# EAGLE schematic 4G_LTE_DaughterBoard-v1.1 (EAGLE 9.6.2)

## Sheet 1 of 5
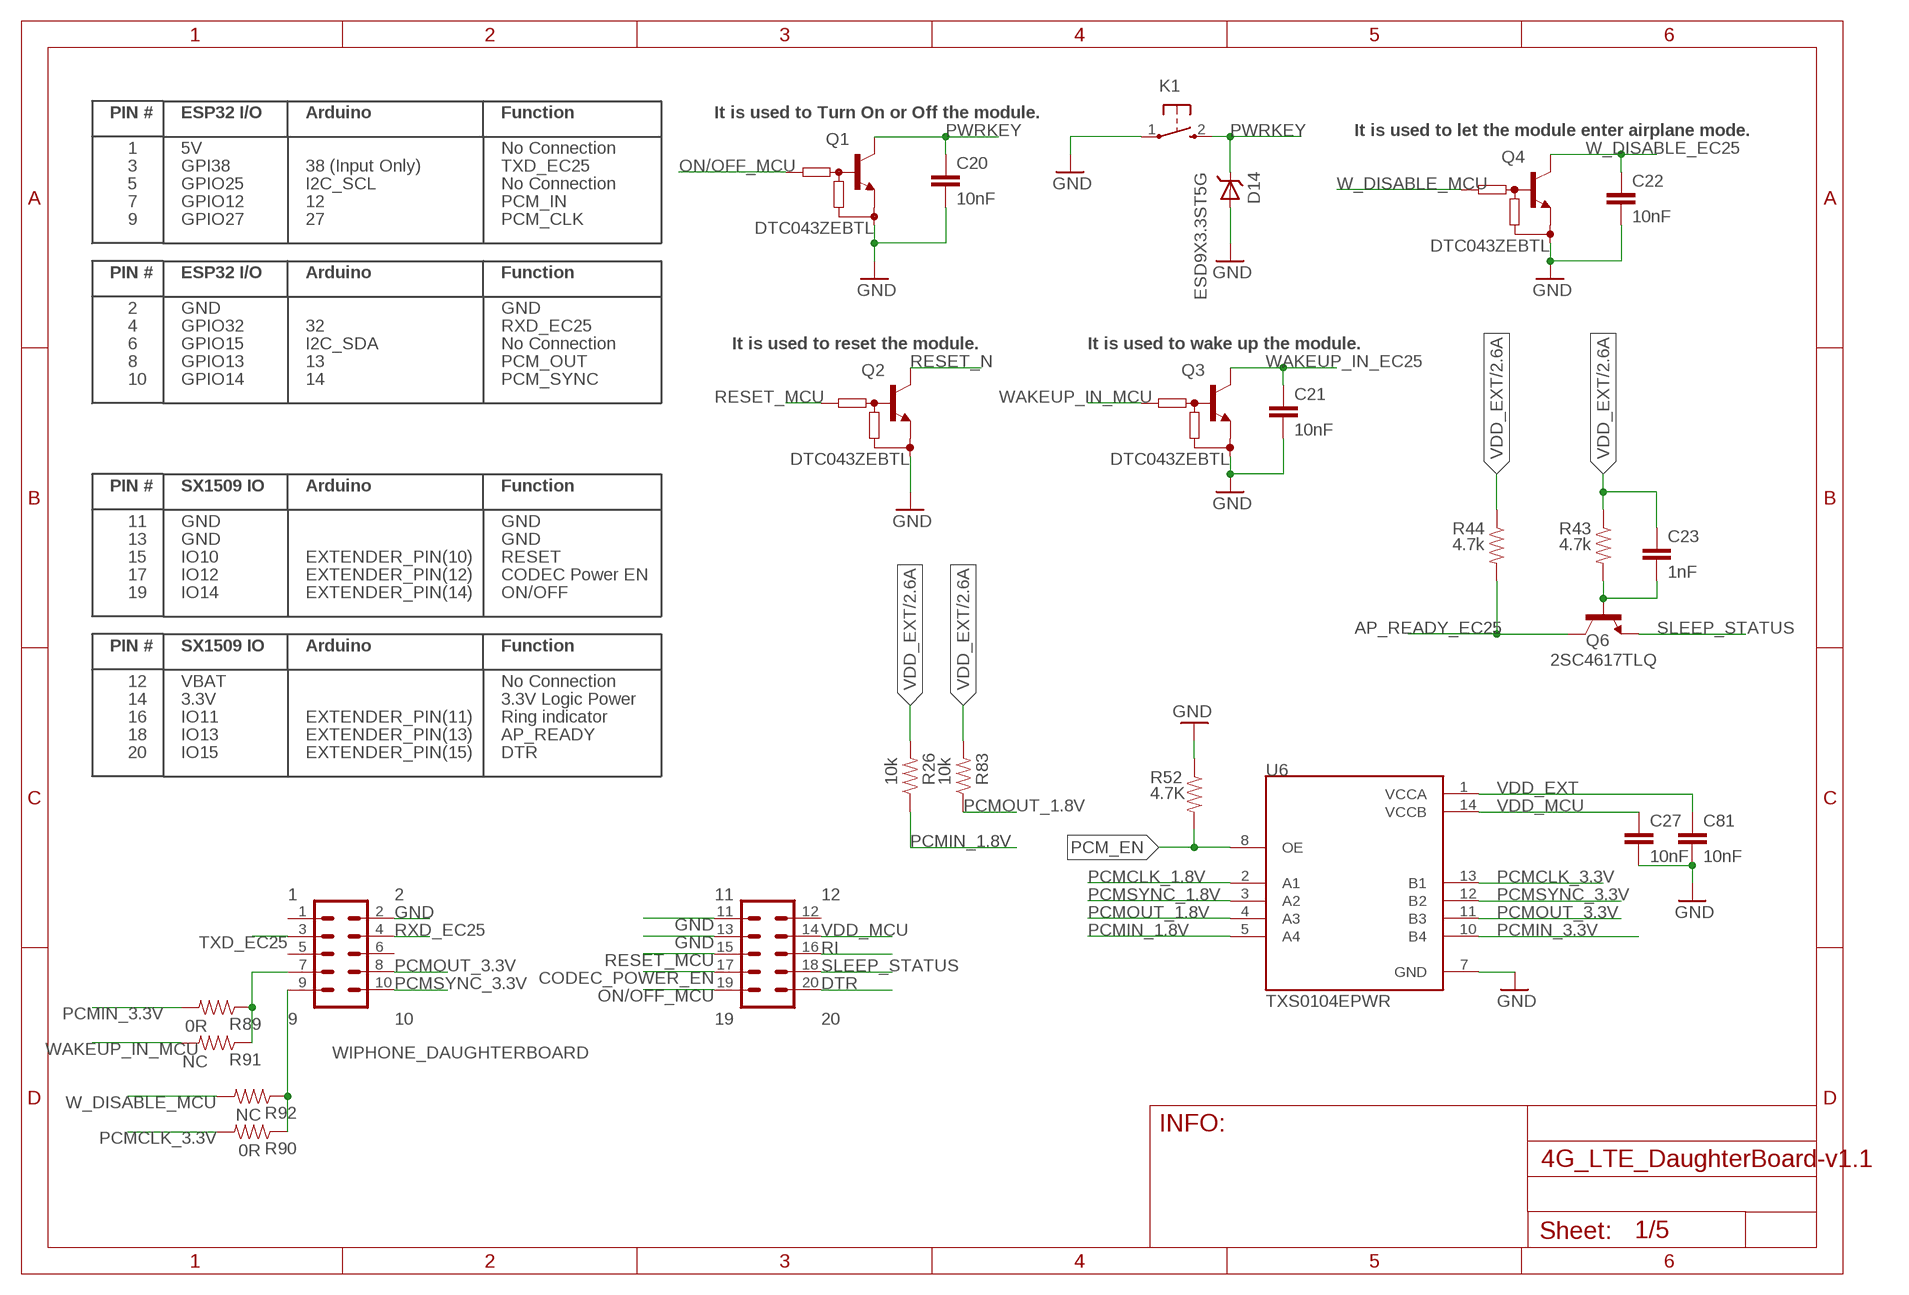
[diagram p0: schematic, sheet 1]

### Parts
C20  10nF  CAP0402  [0402-CAP]
C21  10nF  CAP0402  [0402-CAP]
C22  10nF  CAP0402  [0402-CAP]
C23  1nF  CAP0402  [0402-CAP]
C27  10nF  CAP0402  [0402-CAP]
C81  10nF  CAP0402  [0402-CAP]
D14  ESD9X3.3ST5G  [SODFL1060X40N]
K1  BUTTON_3X6X5-90_DEGREE  [3X6X5-90_DEGREE]
Q1  DTC043ZEBTL  DIGITAL_TRANSISTOR-SC89  [SC89]
Q2  DTC043ZEBTL  DIGITAL_TRANSISTOR-SC89  [SC89]
Q3  DTC043ZEBTL  DIGITAL_TRANSISTOR-SC89  [SC89]
Q4  DTC043ZEBTL  DIGITAL_TRANSISTOR-SC89  [SC89]
Q6  2SC4617TLQ  TRANS_NPN-L  [SOT23-3-L]
R26  10k  RES0402  [0402-RES]
R43  4.7k  RES0402  [0402-RES]
R44  4.7k  RES0402  [0402-RES]
R52  4.7K  RES0402  [0402-RES]
R83  10k  RES0402  [0402-RES]
R89  0R  RES0402  [0402-RES]
R90  0R  RES0402  [0402-RES]
R91  NC  RES0402  [0402-RES]
R92  NC  RES0402  [0402-RES]
U6  TXS0104EPWR  [SOP65P640X120-14N]
WIPHONE_DAUGHTERBOARD-FOOTPRINT1  WIPHONE_DAUGHTERBOARD  [WIPHONE_DAUGHTERBOARD]

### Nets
AP_READY_EC25: Q6.3(C) R44.2 ; also sheet 2
CODEC_POWER_EN: WIPHONE_DAUGHTERBOARD-FOOTPRINT1.17 ; also sheet 5
DTR: WIPHONE_DAUGHTERBOARD-FOOTPRINT1.20 ; also sheet 2
GND: C20.2 C21.2 C22.2 C27.2 C81.2 D14.2 K1.1 Q1.2(E) Q2.2(E) Q3.2(E) Q4.2(E) R52.1 U6.7(GND) WIPHONE_DAUGHTERBOARD-FOOTPRINT1.2 WIPHONE_DAUGHTERBOARD-FOOTPRINT1.11 WIPHONE_DAUGHTERBOARD-FOOTPRINT1.13 ; also sheet 2,3,4,5
N$29: C23.2 Q6.1(B) R43.2
N$73: R89.1 R91.1 WIPHONE_DAUGHTERBOARD-FOOTPRINT1.7
N$74: R90.1 R92.1 WIPHONE_DAUGHTERBOARD-FOOTPRINT1.9
ON/OFF_MCU: Q1.1(B) WIPHONE_DAUGHTERBOARD-FOOTPRINT1.19
PCM_EN: R52.2 U6.8(OE)
PCMCLK_1.8V: U6.2(A1) ; also sheet 2
PCMCLK_3.3V: R90.2 U6.13(B1)
PCMIN_1.8V: R26.1 U6.5(A4) ; also sheet 2
PCMIN_3.3V: R89.2 U6.10(B4)
PCMOUT_1.8V: R83.1 U6.4(A3) ; also sheet 2
PCMOUT_3.3V: U6.11(B3) WIPHONE_DAUGHTERBOARD-FOOTPRINT1.8
PCMSYNC_1.8V: U6.3(A2) ; also sheet 2
PCMSYNC_3.3V: U6.12(B2) WIPHONE_DAUGHTERBOARD-FOOTPRINT1.10
PWRKEY: C20.1 D14.1 K1.2 Q1.3(C) ; also sheet 2
RESET_MCU: Q2.1(B) WIPHONE_DAUGHTERBOARD-FOOTPRINT1.15
RESET_N: Q2.3(C) ; also sheet 2
RI: WIPHONE_DAUGHTERBOARD-FOOTPRINT1.16 ; also sheet 2
RXD_EC25: WIPHONE_DAUGHTERBOARD-FOOTPRINT1.4 ; also sheet 2
SLEEP_STATUS: Q6.2(E) WIPHONE_DAUGHTERBOARD-FOOTPRINT1.18
TXD_EC25: WIPHONE_DAUGHTERBOARD-FOOTPRINT1.3 ; also sheet 2
VDD_EXT: C23.1 C81.1 R26.2 R43.1 R44.1 R83.2 U6.1(VCCA) ; also sheet 2,3,5
VDD_MCU: C27.1 U6.14(VCCB) WIPHONE_DAUGHTERBOARD-FOOTPRINT1.14
W_DISABLE_EC25: C22.1 Q4.3(C) ; also sheet 2
W_DISABLE_MCU: Q4.1(B) R92.2
WAKEUP_IN_EC25: C21.1 Q3.3(C) ; also sheet 2
WAKEUP_IN_MCU: Q3.1(B) R91.2
Unconnected: WIPHONE_DAUGHTERBOARD-FOOTPRINT1.5 WIPHONE_DAUGHTERBOARD-FOOTPRINT1.6

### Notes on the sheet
- It is used to Turn On or Off the module.
- It is used to let the module enter airplane mode.
- No Connection
- TXD_EC25
- No Connection
- PCM_IN
- PCM_CLK
- GND
- RXD_EC25
- No Connection | It is used to reset the module. | It is used to wake up the module.
- PCM_OUT
- PCM_SYNC
- GND
- GND
- RESET
- CODEC Power EN
- ON/OFF
- No Connection
- 3.3V Logic Power
- Ring indicator
- AP_READY
- DTR

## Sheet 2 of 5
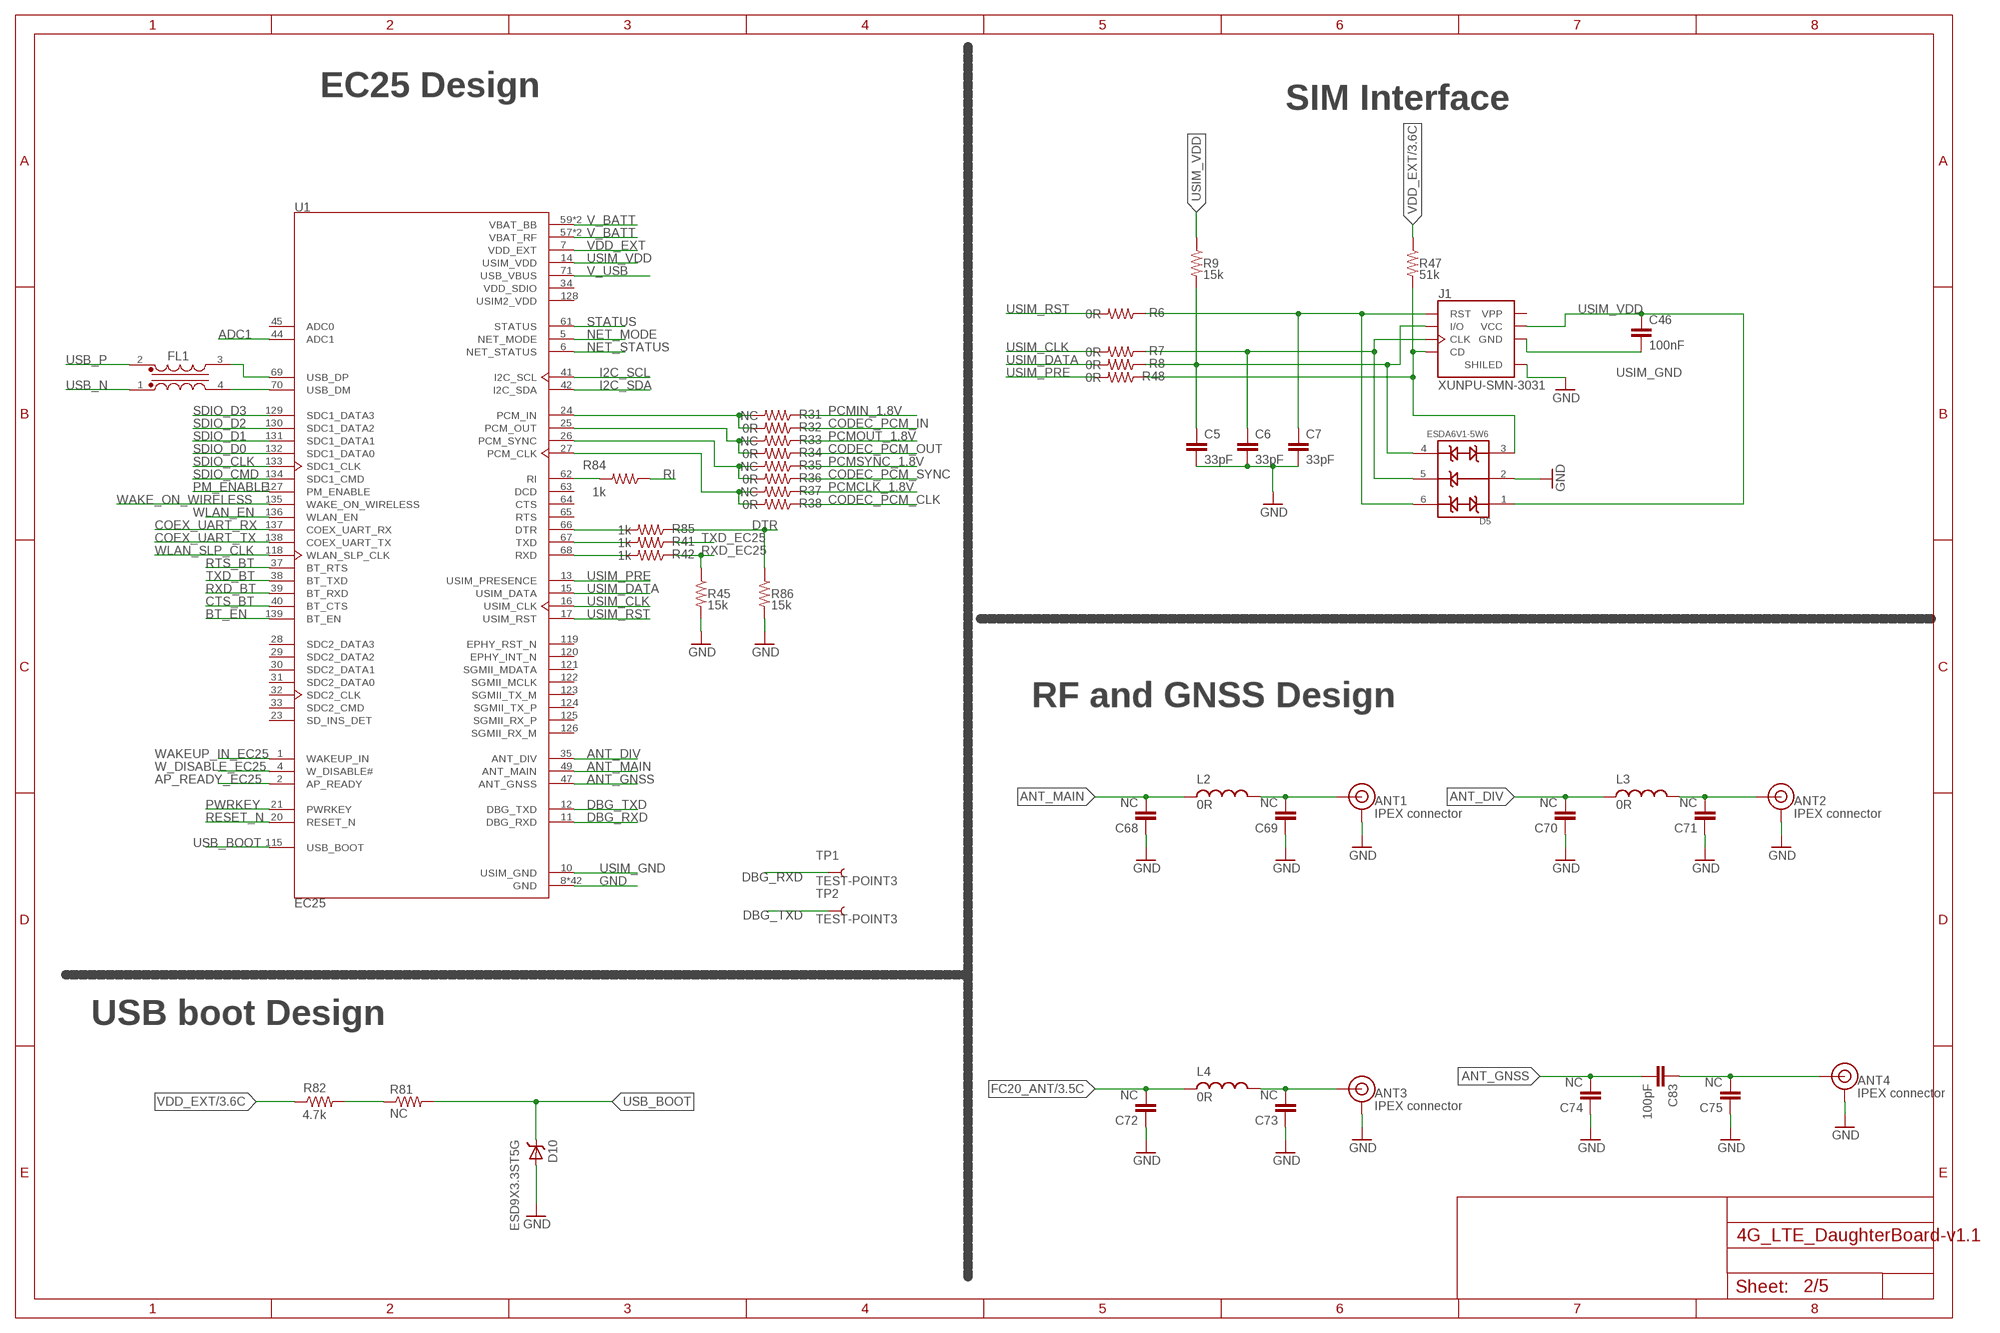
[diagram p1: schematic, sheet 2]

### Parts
ANT1  IPEX connector  U.FL2PIN  [U.FL]
ANT2  IPEX connector  U.FL2PIN  [U.FL]
ANT3  IPEX connector  U.FL2PIN  [U.FL]
ANT4  IPEX connector  U.FL2PIN  [U.FL]
C5  33pF  CAP0402  [0402-CAP]
C6  33pF  CAP0402  [0402-CAP]
C7  33pF  CAP0402  [0402-CAP]
C46  100nF  CAP0402  [0402-CAP]
C68  NC  CAP0402  [0402-CAP]
C69  NC  CAP0402  [0402-CAP]
C70  NC  CAP0402  [0402-CAP]
C71  NC  CAP0402  [0402-CAP]
C72  NC  CAP0402  [0402-CAP]
C73  NC  CAP0402  [0402-CAP]
C74  NC  CAP0402  [0402-CAP]
C75  NC  CAP0402  [0402-CAP]
C83  100pF  CAP0402  [0402-CAP]
D5  ESDA6V1-5W6  [DIO_ESDA6V1-5W6]
D10  ESD9X3.3ST5G  [SODFL1060X40N]
FL1  CHOKE  [SMD,1.25X1.0X0.5MM]
J1  XUNPU-SMN-3031  [XUNPU-SMN-303_C266888]
L2  0R  IND0402  [0402-IND]
L3  0R  IND0402  [0402-IND]
L4  0R  IND0402  [0402-IND]
R6  0R  RES0402  [0402-RES]
R7  0R  RES0402  [0402-RES]
R8  0R  RES0402  [0402-RES]
R9  15k  RES0402  [0402-RES]
R31  NC  RES0402  [0402-RES]
R32  0R  RES0402  [0402-RES]
R33  NC  RES0402  [0402-RES]
R34  0R  RES0402  [0402-RES]
R35  NC  RES0402  [0402-RES]
R36  0R  RES0402  [0402-RES]
R37  NC  RES0402  [0402-RES]
R38  0R  RES0402  [0402-RES]
R41  1k  RES0402  [0402-RES]
R42  1k  RES0402  [0402-RES]
R45  15k  RES0402  [0402-RES]
R47  51k  RES0402  [0402-RES]
R48  0R  RES0402  [0402-RES]
R81  NC  RES0402  [0402-RES]
R82  4.7k  RES0402  [0402-RES]
R84  1k  RES0402  [0402-RES]
R85  1k  RES0402  [0402-RES]
R86  15k  RES0402  [0402-RES]
TP1  TEST-POINT3  [PAD.03X.03]
TP2  TEST-POINT3  [PAD.03X.03]
U1  EC25  [EC25EFA]

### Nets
ADC1: U1.44(ADC1)
ANT_DIV: C70.2 L3.1 U1.35(ANT_DIV)
ANT_GNSS: C74.2 C83.2 U1.47(ANT_GNSS)
ANT_MAIN: C68.2 L2.1 U1.49(ANT_MAIN)
AP_READY_EC25: U1.2(AP_READY) ; also sheet 1
BT_EN: U1.139(BT_EN) ; also sheet 3
CODEC_PCM_CLK: R38.1 ; also sheet 4
CODEC_PCM_IN: R32.1 ; also sheet 4
CODEC_PCM_OUT: R34.1 ; also sheet 4
CODEC_PCM_SYNC: R36.1 ; also sheet 4
COEX_UART_RX: U1.137(COEX_UART_RX) ; also sheet 3
COEX_UART_TX: U1.138(COEX_UART_TX) ; also sheet 3
CTS_BT: U1.40(BT_CTS) ; also sheet 3
DBG_RXD: TP1.P$1 U1.11(DBG_RXD)
DBG_TXD: TP2.P$1 U1.12(DBG_TXD)
DTR: R85.1 R86.1 ; also sheet 1
FC20_ANT: C72.2 L4.1 ; also sheet 3
GND: ANT1.1(GND) ANT1.2(GND) ANT2.1(GND) ANT2.2(GND) ANT3.1(GND) ANT3.2(GND) ANT4.1(GND) ANT4.2(GND) C5.2 C6.2 C7.2 C68.1 C69.1 C70.1 C71.1 C72.1 C73.1 C74.1 C75.1 D5.2 D10.2 J1.P$1(SHILED) J1.P$2(SHILED) J1.P$3(SHILED) J1.P$4(SHILED) R45.2 R86.2 U1.8(GND) U1.9(GND) U1.19(GND) U1.22(GND) U1.36(GND) U1.46(GND) U1.48(GND) U1.50(GND) U1.51(GND) U1.52(GND) U1.53(GND) U1.54(GND) U1.56(GND) U1.72(GND) U1.85(GND) U1.86(GND) U1.87(GND) U1.88(GND) U1.89(GND) U1.90(GND) U1.91(GND) U1.92(GND) U1.93(GND) U1.94(GND) U1.95(GND) U1.96(GND) U1.97(GND) U1.98(GND) U1.99(GND) U1.100(GND) U1.101(GND) U1.102(GND) U1.103(GND) U1.104(GND) U1.105(GND) U1.106(GND) U1.107(GND) U1.108(GND) U1.109(GND) U1.110(GND) U1.111(GND) U1.112(GND) ; also sheet 1,3,4,5
I2C_SCL: U1.41(I2C_SCL) ; also sheet 4
I2C_SDA: U1.42(I2C_SDA) ; also sheet 4
N$12: R31.2 R32.2 U1.24(PCM_IN)
N$14: R33.2 R34.2 U1.25(PCM_OUT)
N$15: R41.2 U1.67(TXD)
N$16: R35.2 R36.2 U1.26(PCM_SYNC)
N$17: R42.2 U1.68(RXD)
N$18: R37.2 R38.2 U1.27(PCM_CLK)
N$19: R81.1 R82.2
N$21: FL1.3 U1.69(USB_DP)
N$26: FL1.4 U1.70(USB_DM)
N$35: C5.1 D5.4 J1.C7(I/O) R8.1 R9.2
N$36: C6.1 D5.5 J1.C3(CLK) R7.1
N$37: C7.1 D5.6 J1.C2(RST) R6.1
N$57: ANT2.FEED(SIGNAL) C71.2 L3.2
N$58: ANT3.FEED(SIGNAL) C73.2 L4.2
N$59: ANT4.FEED(SIGNAL) C75.2 C83.1
N$61: ANT1.FEED(SIGNAL) C69.2 L2.2
N$66: R84.2 U1.62(RI)
N$69: D5.3 J1.CD R47.2 R48.1
N$71: R85.2 U1.66(DTR)
NET_MODE: U1.5(NET_MODE) ; also sheet 5
NET_STATUS: U1.6(NET_STATUS) ; also sheet 5
PCMCLK_1.8V: R37.1 ; also sheet 1
PCMIN_1.8V: R31.1 ; also sheet 1
PCMOUT_1.8V: R33.1 ; also sheet 1
PCMSYNC_1.8V: R35.1 ; also sheet 1
PM_ENABLE: U1.127(PM_ENABLE) ; also sheet 5
PWRKEY: U1.21(PWRKEY) ; also sheet 1
RESET_N: U1.20(RESET_N) ; also sheet 1
RI: R84.1 ; also sheet 1
RTS_BT: U1.37(BT_RTS) ; also sheet 3
RXD_BT: U1.39(BT_RXD) ; also sheet 3
RXD_EC25: R42.1 R45.1 ; also sheet 1
SDIO_CLK: U1.133(SDC1_CLK) ; also sheet 3
SDIO_CMD: U1.134(SDC1_CMD) ; also sheet 3
SDIO_D0: U1.132(SDC1_DATA0) ; also sheet 3
SDIO_D1: U1.131(SDC1_DATA1) ; also sheet 3
SDIO_D2: U1.130(SDC1_DATA2) ; also sheet 3
SDIO_D3: U1.129(SDC1_DATA3) ; also sheet 3
STATUS: U1.61(STATUS) ; also sheet 5
TXD_BT: U1.38(BT_TXD) ; also sheet 3
TXD_EC25: R41.1 ; also sheet 1
USB_BOOT: D10.1 R81.2 U1.115(USB_BOOT)
USB_N [USB_Data]: FL1.1 ; also sheet 5
USB_P [USB_Data]: FL1.2 ; also sheet 5
USIM_CLK: R7.2 U1.16(USIM_CLK)
USIM_DATA: R8.2 U1.15(USIM_DATA)
USIM_GND: C46.2 J1.C5(GND) U1.10(USIM_GND)
USIM_PRE: R48.2 U1.13(USIM_PRESENCE)
USIM_RST: R6.2 U1.17(USIM_RST)
USIM_VDD: C46.1 D5.1 J1.C1(VCC) R9.1 U1.14(USIM_VDD)
V_BATT: U1.57(VBAT_RF) U1.58(VBAT_RF) U1.59(VBAT_BB) U1.60(VBAT_BB) ; also sheet 5
V_USB: U1.71(USB_VBUS) ; also sheet 5
VDD_EXT: R47.1 R82.1 U1.7(VDD_EXT) ; also sheet 1,3,5
W_DISABLE_EC25: U1.4(W_DISABLE#) ; also sheet 1
WAKE_ON_WIRELESS: U1.135(WAKE_ON_WIRELESS) ; also sheet 3
WAKEUP_IN_EC25: U1.1(WAKEUP_IN) ; also sheet 1
WLAN_EN: U1.136(WLAN_EN) ; also sheet 3
WLAN_SLP_CLK: U1.118(WLAN_SLP_CLK) ; also sheet 3
Unconnected: U1.23(SD_INS_DET) U1.28(SDC2_DATA3) U1.29(SDC2_DATA2) U1.30(SDC2_DATA1) U1.31(SDC2_DATA0) U1.32(SDC2_CLK) U1.33(SDC2_CMD) U1.45(ADC0) U1.63(DCD) U1.64(CTS) U1.65(RTS) U1.119(EPHY_RST_N) U1.120(EPHY_INT_N) U1.121(SGMII_MDATA) U1.122(SGMII_MCLK) U1.123(SGMII_TX_M) U1.124(SGMII_TX_P) U1.125(SGMII_RX_P) U1.126(SGMII_RX_M)

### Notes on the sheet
- EC25 Design
- SIM Interface
- RF and GNSS Design
- USB boot Design

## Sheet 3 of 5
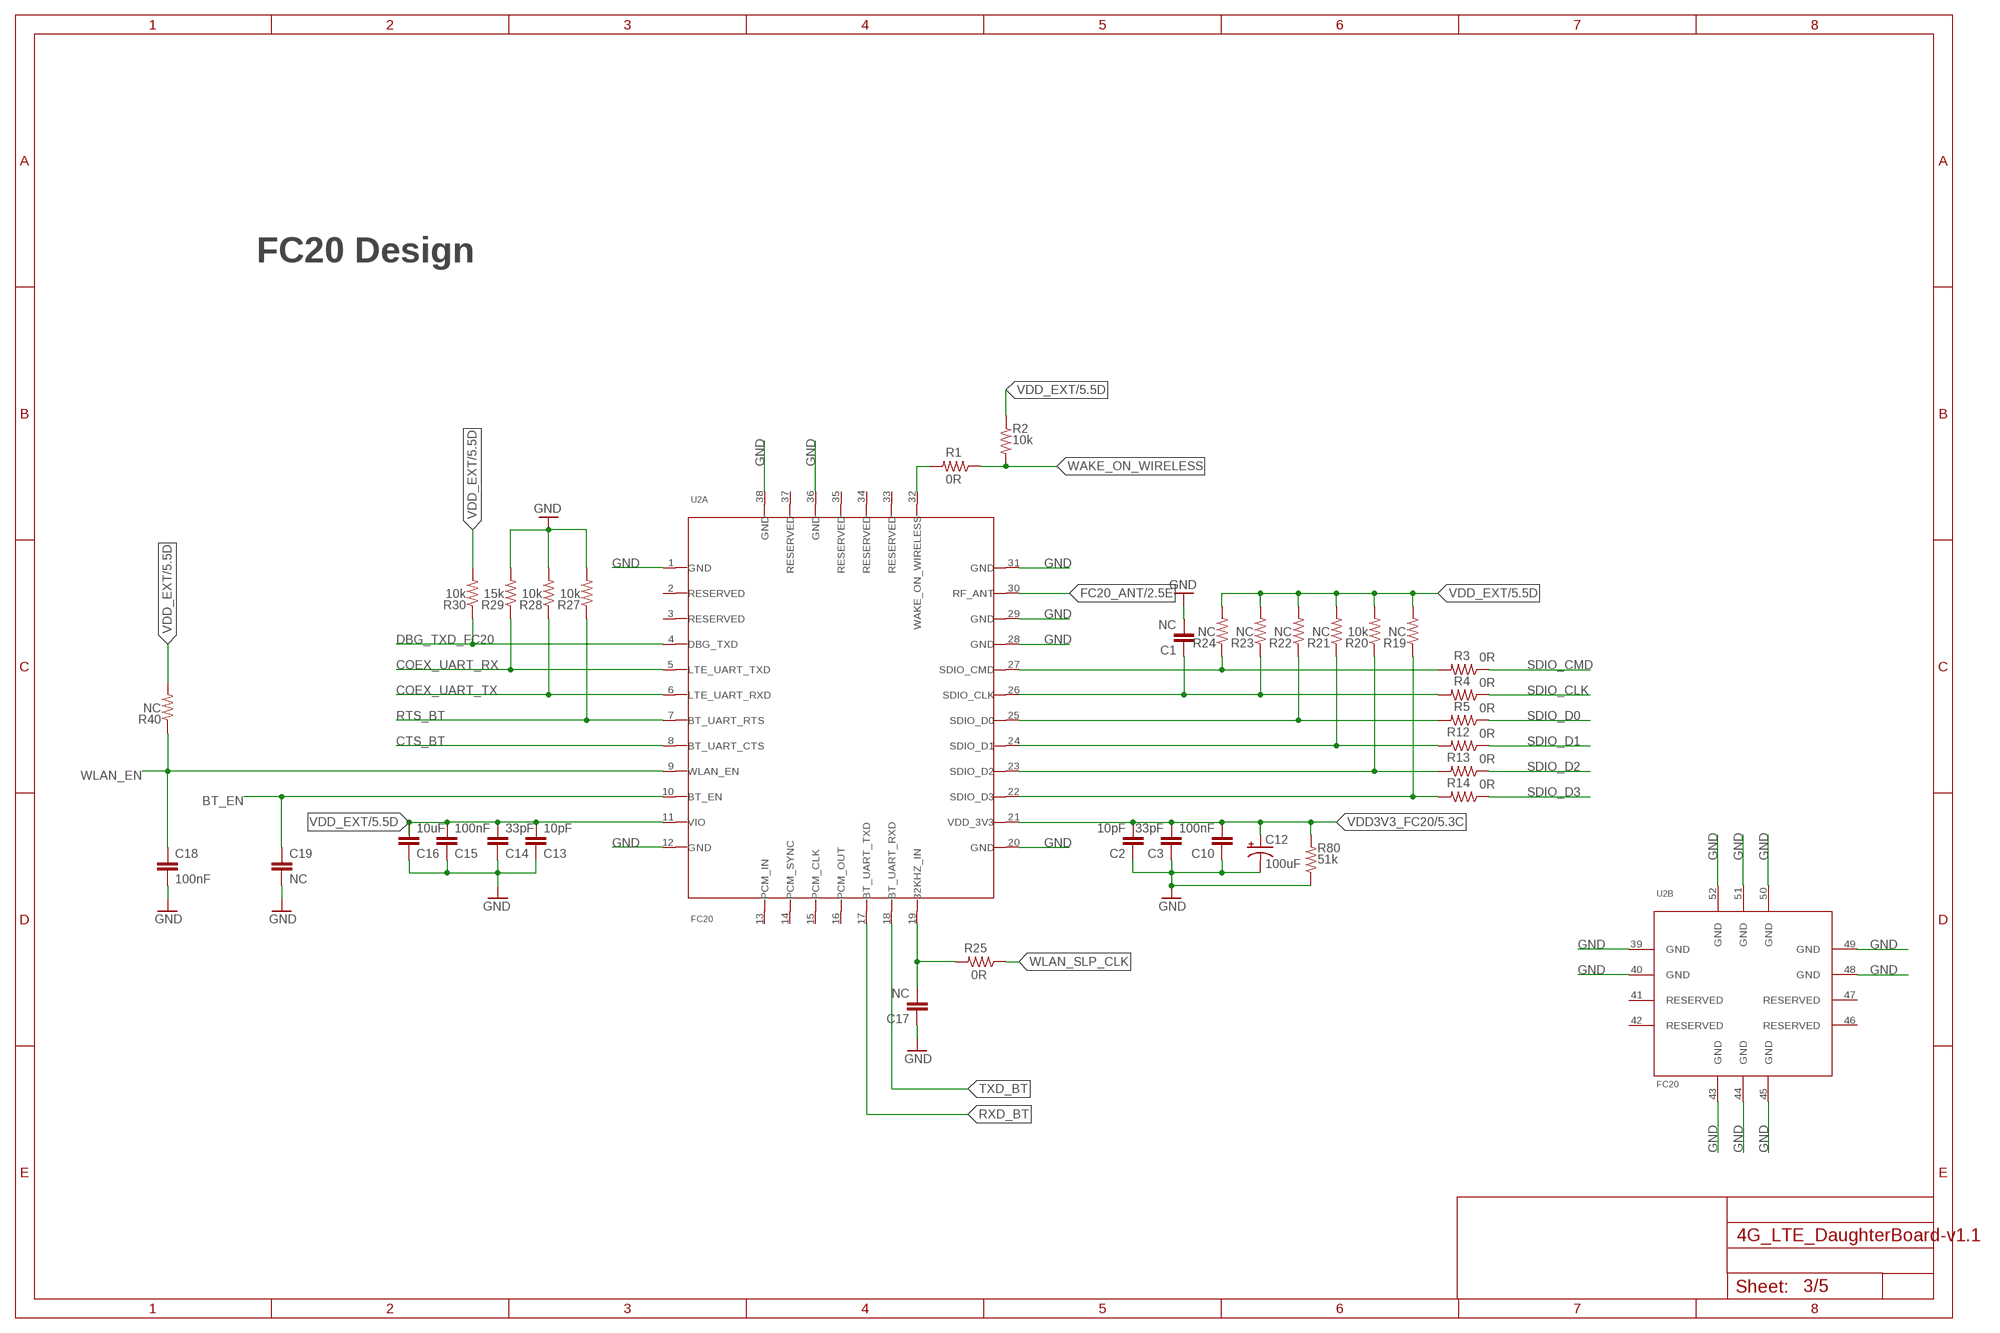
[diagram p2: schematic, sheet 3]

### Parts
C1  NC  CAP0402  [0402-CAP]
C2  10pF  CAP0402  [0402-CAP]
C3  33pF  CAP0402  [0402-CAP]
C10  100nF  CAP0402  [0402-CAP]
C12  100uF  CAP_TANT_AVX-B  [AVX-B]
C13  10pF  CAP0402  [0402-CAP]
C14  33pF  CAP0402  [0402-CAP]
C15  100nF  CAP0402  [0402-CAP]
C16  10uF  CAP0402  [0402-CAP]
C17  NC  CAP0402  [0402-CAP]
C18  100nF  CAP0402  [0402-CAP]
C19  NC  CAP0402  [0402-CAP]
R1  0R  RES0402  [0402-RES]
R2  10k  RES0402  [0402-RES]
R3  0R  RES0402  [0402-RES]
R4  0R  RES0402  [0402-RES]
R5  0R  RES0402  [0402-RES]
R12  0R  RES0402  [0402-RES]
R13  0R  RES0402  [0402-RES]
R14  0R  RES0402  [0402-RES]
R19  NC  RES0402  [0402-RES]
R20  10k  RES0402  [0402-RES]
R21  NC  RES0402  [0402-RES]
R22  NC  RES0402  [0402-RES]
R23  NC  RES0402  [0402-RES]
R24  NC  RES0402  [0402-RES]
R25  0R  RES0402  [0402-RES]
R27  10k  RES0402  [0402-RES]
R28  10k  RES0402  [0402-RES]
R29  15k  RES0402  [0402-RES]
R30  10k  RES0402  [0402-RES]
R40  NC  RES0402  [0402-RES]
R80  51k  RES0402  [0402-RES]
U2  FC20  [FC20N]

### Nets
BT_EN: C19.1 U2.10(A:BT_EN) ; also sheet 2
COEX_UART_RX: R29.1 U2.5(A:LTE_UART_TXD) ; also sheet 2
COEX_UART_TX: R28.1 U2.6(A:LTE_UART_RXD) ; also sheet 2
CTS_BT: U2.8(A:BT_UART_CTS) ; also sheet 2
DBG_TXD_FC20: R30.1 U2.4(A:DBG_TXD)
FC20_ANT: U2.30(A:RF_ANT) ; also sheet 2
GND: C1.2 C2.1 C3.1 C10.1 C12.- C13.1 C14.1 C15.1 C16.1 C17.1 C18.2 C19.2 R27.2 R28.2 R29.2 R80.1 U2.1(A:GND) U2.12(A:GND) U2.20(A:GND) U2.28(A:GND) U2.29(A:GND) U2.31(A:GND) U2.36(A:GND) U2.38(A:GND) U2.39(B:GND) U2.40(B:GND) U2.43(B:GND) U2.44(B:GND) U2.45(B:GND) U2.48(B:GND) U2.49(B:GND) U2.50(B:GND) U2.51(B:GND) U2.52(B:GND) ; also sheet 1,2,4,5
N$4: R1.2 U2.32(A:WAKE_ON_WIRELESS)
N$5: R3.2 R24.1 U2.27(A:SDIO_CMD)
N$6: C1.1 R4.2 R23.1 U2.26(A:SDIO_CLK)
N$7: R5.2 R22.1 U2.25(A:SDIO_D0)
N$8: R12.2 R21.1 U2.24(A:SDIO_D1)
N$9: R13.2 R20.1 U2.23(A:SDIO_D2)
N$10: R14.2 R19.1 U2.22(A:SDIO_D3)
N$11: C17.2 R25.2 U2.19(A:32KHZ_IN)
RTS_BT: R27.1 U2.7(A:BT_UART_RTS) ; also sheet 2
RXD_BT: U2.17(A:BT_UART_TXD) ; also sheet 2
SDIO_CLK: R4.1 ; also sheet 2
SDIO_CMD: R3.1 ; also sheet 2
SDIO_D0: R5.1 ; also sheet 2
SDIO_D1: R12.1 ; also sheet 2
SDIO_D2: R13.1 ; also sheet 2
SDIO_D3: R14.1 ; also sheet 2
TXD_BT: U2.18(A:BT_UART_RXD) ; also sheet 2
VDD3V3_FC20: C2.2 C3.2 C10.2 C12.+ R80.2 U2.21(A:VDD_3V3) ; also sheet 5
VDD_EXT: C13.2 C14.2 C15.2 C16.2 R2.1 R19.2 R20.2 R21.2 R22.2 R23.2 R24.2 R30.2 R40.2 U2.11(A:VIO) ; also sheet 1,2,5
WAKE_ON_WIRELESS: R1.1 R2.2 ; also sheet 2
WLAN_EN: C18.1 R40.1 U2.9(A:WLAN_EN) ; also sheet 2
WLAN_SLP_CLK: R25.1 ; also sheet 2
Unconnected: U2.2(A:RESERVED) U2.3(A:RESERVED) U2.13(A:PCM_IN) U2.14(A:PCM_SYNC) U2.15(A:PCM_CLK) U2.16(A:PCM_OUT) U2.33(A:RESERVED) U2.34(A:RESERVED) U2.35(A:RESERVED) U2.37(A:RESERVED) U2.41(B:RESERVED) U2.42(B:RESERVED) U2.46(B:RESERVED) U2.47(B:RESERVED)

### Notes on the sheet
- FC20 Design

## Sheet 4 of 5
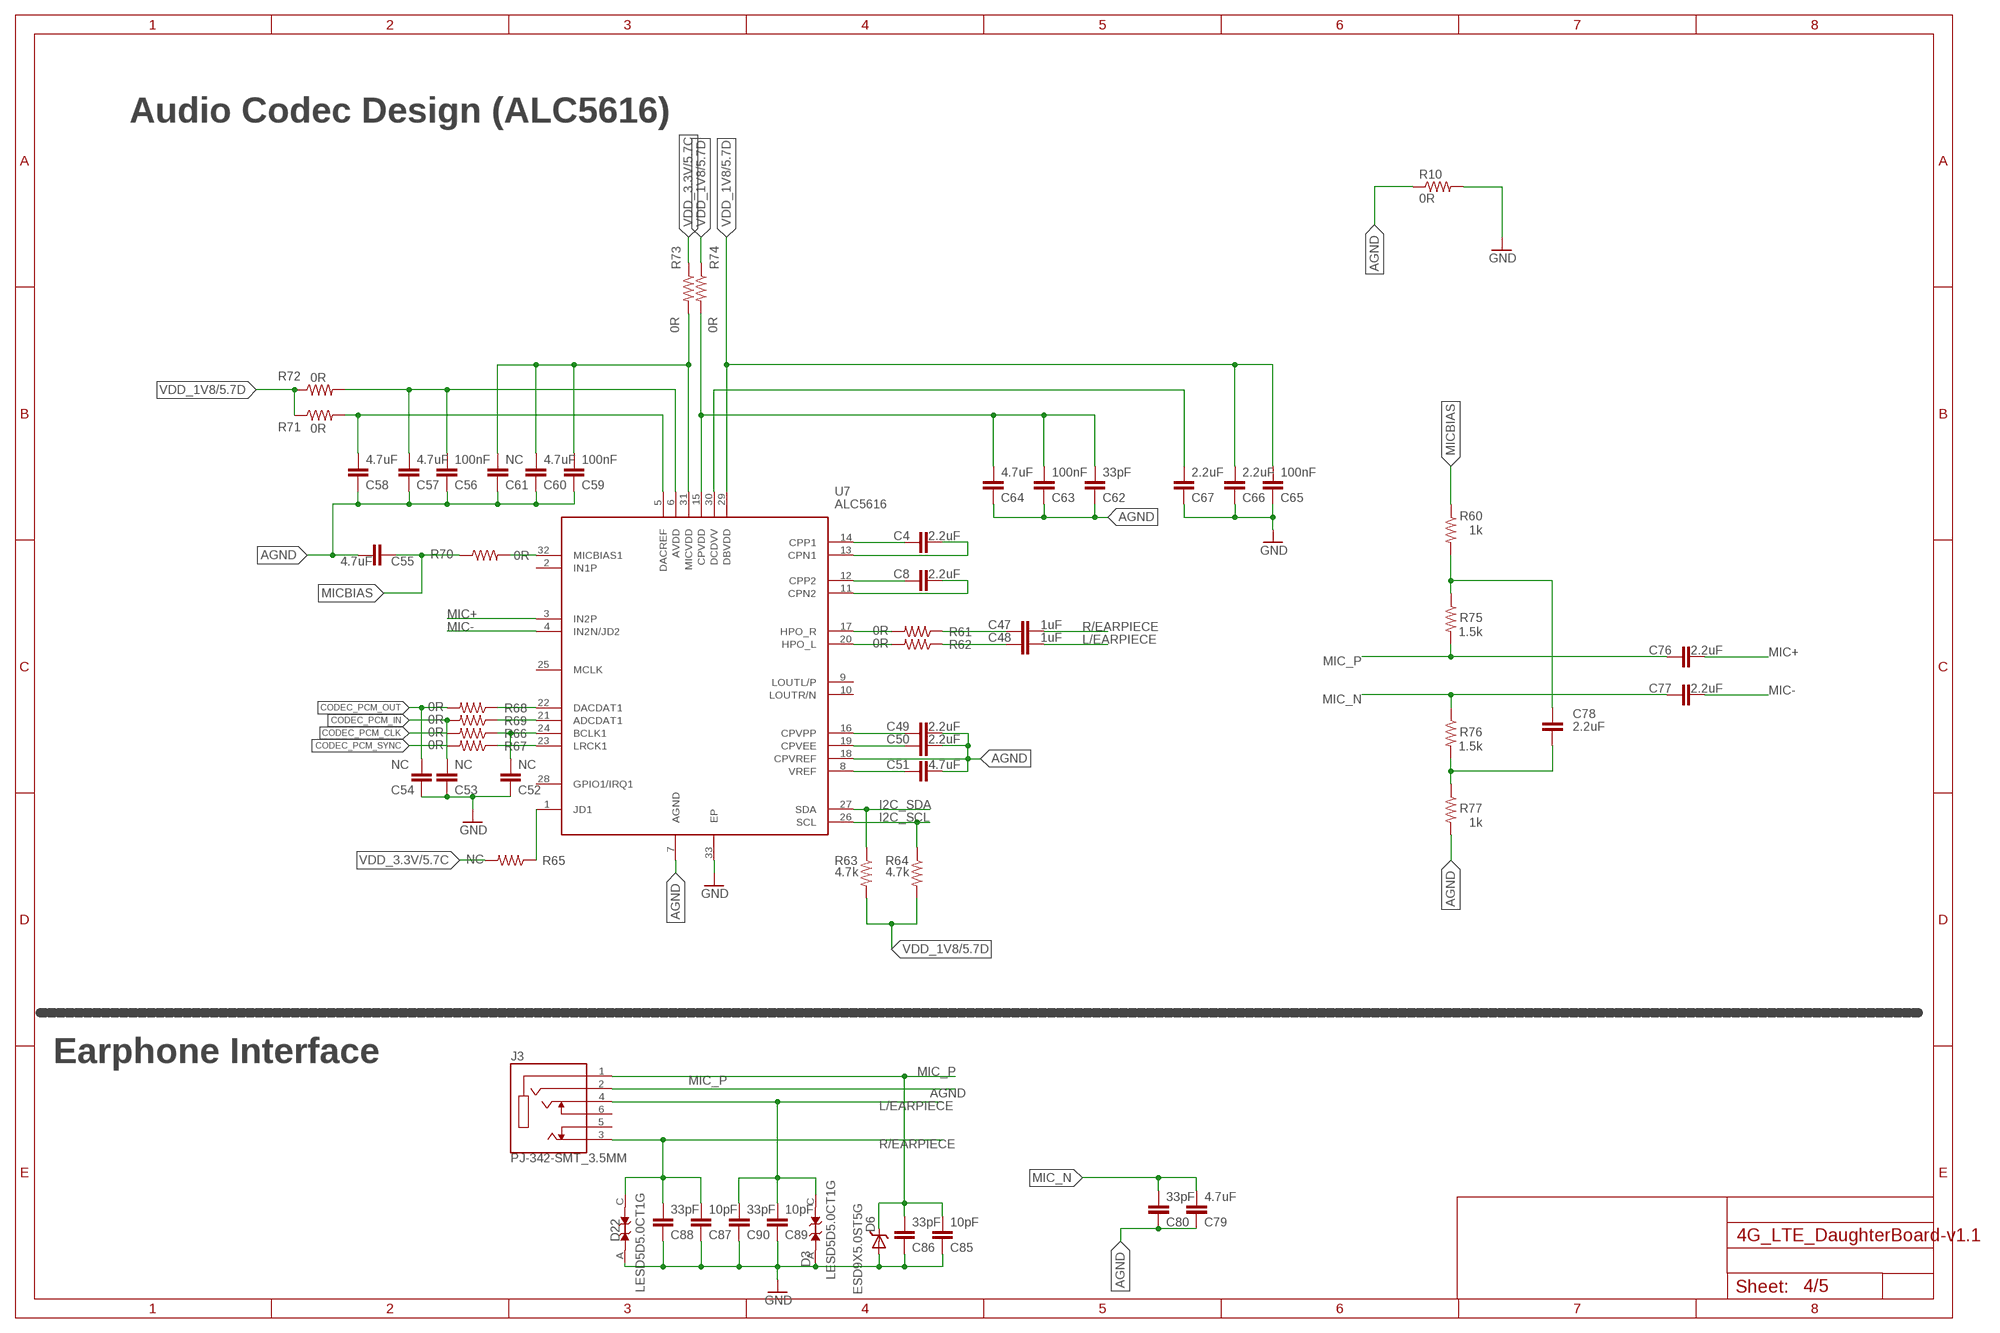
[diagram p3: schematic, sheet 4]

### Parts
C4  2.2uF  CAP0402  [0402-CAP]
C8  2.2uF  CAP0402  [0402-CAP]
C47  1uF  CAP0402  [0402-CAP]
C48  1uF  CAP0402  [0402-CAP]
C49  2.2uF  CAP0402  [0402-CAP]
C50  2.2uF  CAP0402  [0402-CAP]
C51  4.7uF  CAP0402  [0402-CAP]
C52  NC  CAP0402  [0402-CAP]
C53  NC  CAP0402  [0402-CAP]
C54  NC  CAP0402  [0402-CAP]
C55  4.7uF  CAP0402  [0402-CAP]
C56  100nF  CAP0402  [0402-CAP]
C57  4.7uF  CAP0402  [0402-CAP]
C58  4.7uF  CAP0402  [0402-CAP]
C59  100nF  CAP0402  [0402-CAP]
C60  4.7uF  CAP0402  [0402-CAP]
C61  NC  CAP0402  [0402-CAP]
C62  33pF  CAP0402  [0402-CAP]
C63  100nF  CAP0402  [0402-CAP]
C64  4.7uF  CAP0402  [0402-CAP]
C65  100nF  CAP0402  [0402-CAP]
C66  2.2uF  CAP0402  [0402-CAP]
C67  2.2uF  CAP0402  [0402-CAP]
C76  2.2uF  CAP0402  [0402-CAP]
C77  2.2uF  CAP0402  [0402-CAP]
C78  2.2uF  CAP0402  [0402-CAP]
C79  4.7uF  CAP0402  [0402-CAP]
C80  33pF  CAP0402  [0402-CAP]
C85  10pF  CAP0402  [0402-CAP]
C86  33pF  CAP0402  [0402-CAP]
C87  10pF  CAP0402  [0402-CAP]
C88  33pF  CAP0402  [0402-CAP]
C89  10pF  CAP0402  [0402-CAP]
C90  33pF  CAP0402  [0402-CAP]
D3  LESD5D5.0CT1G  [SOD523]
D6  ESD9X5.0ST5G  ESD9M5.0ST5G  [SODFL1060X40N]
D22  LESD5D5.0CT1G  [SOD523]
J3  PJ-342-SMT_3.5MM  [PJ-342-SMT_3.5MM]
R10  0R  RES0805  [0805_RES]
R60  1k  RES0402  [0402-RES]
R61  0R  RES0402  [0402-RES]
R62  0R  RES0402  [0402-RES]
R63  4.7k  RES0402  [0402-RES]
R64  4.7k  RES0402  [0402-RES]
R65  NC  RES0402  [0402-RES]
R66  0R  RES0402  [0402-RES]
R67  0R  RES0402  [0402-RES]
R68  0R  RES0402  [0402-RES]
R69  0R  RES0402  [0402-RES]
R70  0R  RES0402  [0402-RES]
R71  0R  RES0402  [0402-RES]
R72  0R  RES0402  [0402-RES]
R73  0R  RES0402  [0402-RES]
R74  0R  RES0402  [0402-RES]
R75  1.5k  RES0402  [0402-RES]
R76  1.5k  RES0402  [0402-RES]
R77  1k  RES0402  [0402-RES]
U7  ALC5616  [QFN40P400X400X90-33N]

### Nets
AGND: C49.2 C50.2 C51.2 C55.2 C56.1 C57.1 C58.1 C59.1 C60.1 C61.1 C62.1 C63.1 C64.1 C79.1 C80.1 J3.2 R10.1 R77.2 U7.7(AGND) U7.18(CPVREF)
CODEC_PCM_CLK: R66.2 ; also sheet 2
CODEC_PCM_IN: C53.2 R69.2 ; also sheet 2
CODEC_PCM_OUT: C54.2 R68.2 ; also sheet 2
CODEC_PCM_SYNC: R67.2 ; also sheet 2
GND: C52.1 C53.1 C54.1 C65.1 C66.1 C67.1 C85.1 C86.1 C87.1 C88.1 C89.1 C90.1 D3.A D6.2 D22.A R10.2 U7.33(EP) ; also sheet 1,2,3,5
I2C_SCL: R64.1 U7.26(SCL) ; also sheet 2
I2C_SDA: R63.1 U7.27(SDA) ; also sheet 2
L/EARPIECE: C48.2 C89.2 C90.2 D3.C(A1) J3.4
MIC+: C76.2 U7.3(IN2P)
MIC-: C77.2 U7.4(IN2N/JD2)
MIC_N: C77.1 C79.2 C80.2 R76.1
MIC_P: C76.1 C85.2 C86.2 D6.1 J3.1 R75.2
MICBIAS: C55.1 R60.1 R70.1
N$1: C4.1 U7.14(CPP1)
N$2: C4.2 U7.13(CPN1)
N$3: C8.1 U7.12(CPP2)
N$38: C8.2 U7.11(CPN2)
N$39: R61.2 U7.17(HPO_R)
N$40: R62.2 U7.20(HPO_L)
N$41: C47.1 R61.1
N$42: C48.1 R62.1
N$43: C49.1 U7.16(CPVPP)
N$44: C50.1 U7.19(CPVEE)
N$45: C51.1 U7.8(VREF)
N$46: R65.1 U7.1(JD1)
N$47: R68.1 U7.22(DACDAT1)
N$48: R69.1 U7.21(ADCDAT1)
N$49: C52.2 R66.1 U7.24(BCLK1)
N$50: R67.1 U7.23(LRCK1)
N$51: R70.2 U7.32(MICBIAS1)
N$52: C62.2 C63.2 C64.2 R74.2 U7.15(CPVDD)
N$53: C58.2 R71.2 U7.5(DACREF)
N$54: C56.2 C57.2 R72.2 U7.6(AVDD)
N$55: C67.2 U7.30(DCDVV)
N$56: C59.2 C60.2 C61.2 R73.2 U7.31(MICVDD)
N$60: C78.1 R76.2 R77.1
N$64: C78.2 R60.2 R75.1
R/EARPIECE: C47.2 C87.2 C88.2 D22.C(A1) J3.3
VDD_1V8: C65.2 C66.2 R63.2 R64.2 R71.1 R72.1 R74.1 U7.29(DBVDD) ; also sheet 5
VDD_3.3V: R65.2 R73.1 ; also sheet 5
Unconnected: J3.5 J3.6 U7.2(IN1P) U7.9(LOUTL/P) U7.10(LOUTR/N) U7.25(MCLK) U7.28(GPIO1/IRQ1)

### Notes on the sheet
- Audio Codec Design (ALC5616)
- Earphone Interface

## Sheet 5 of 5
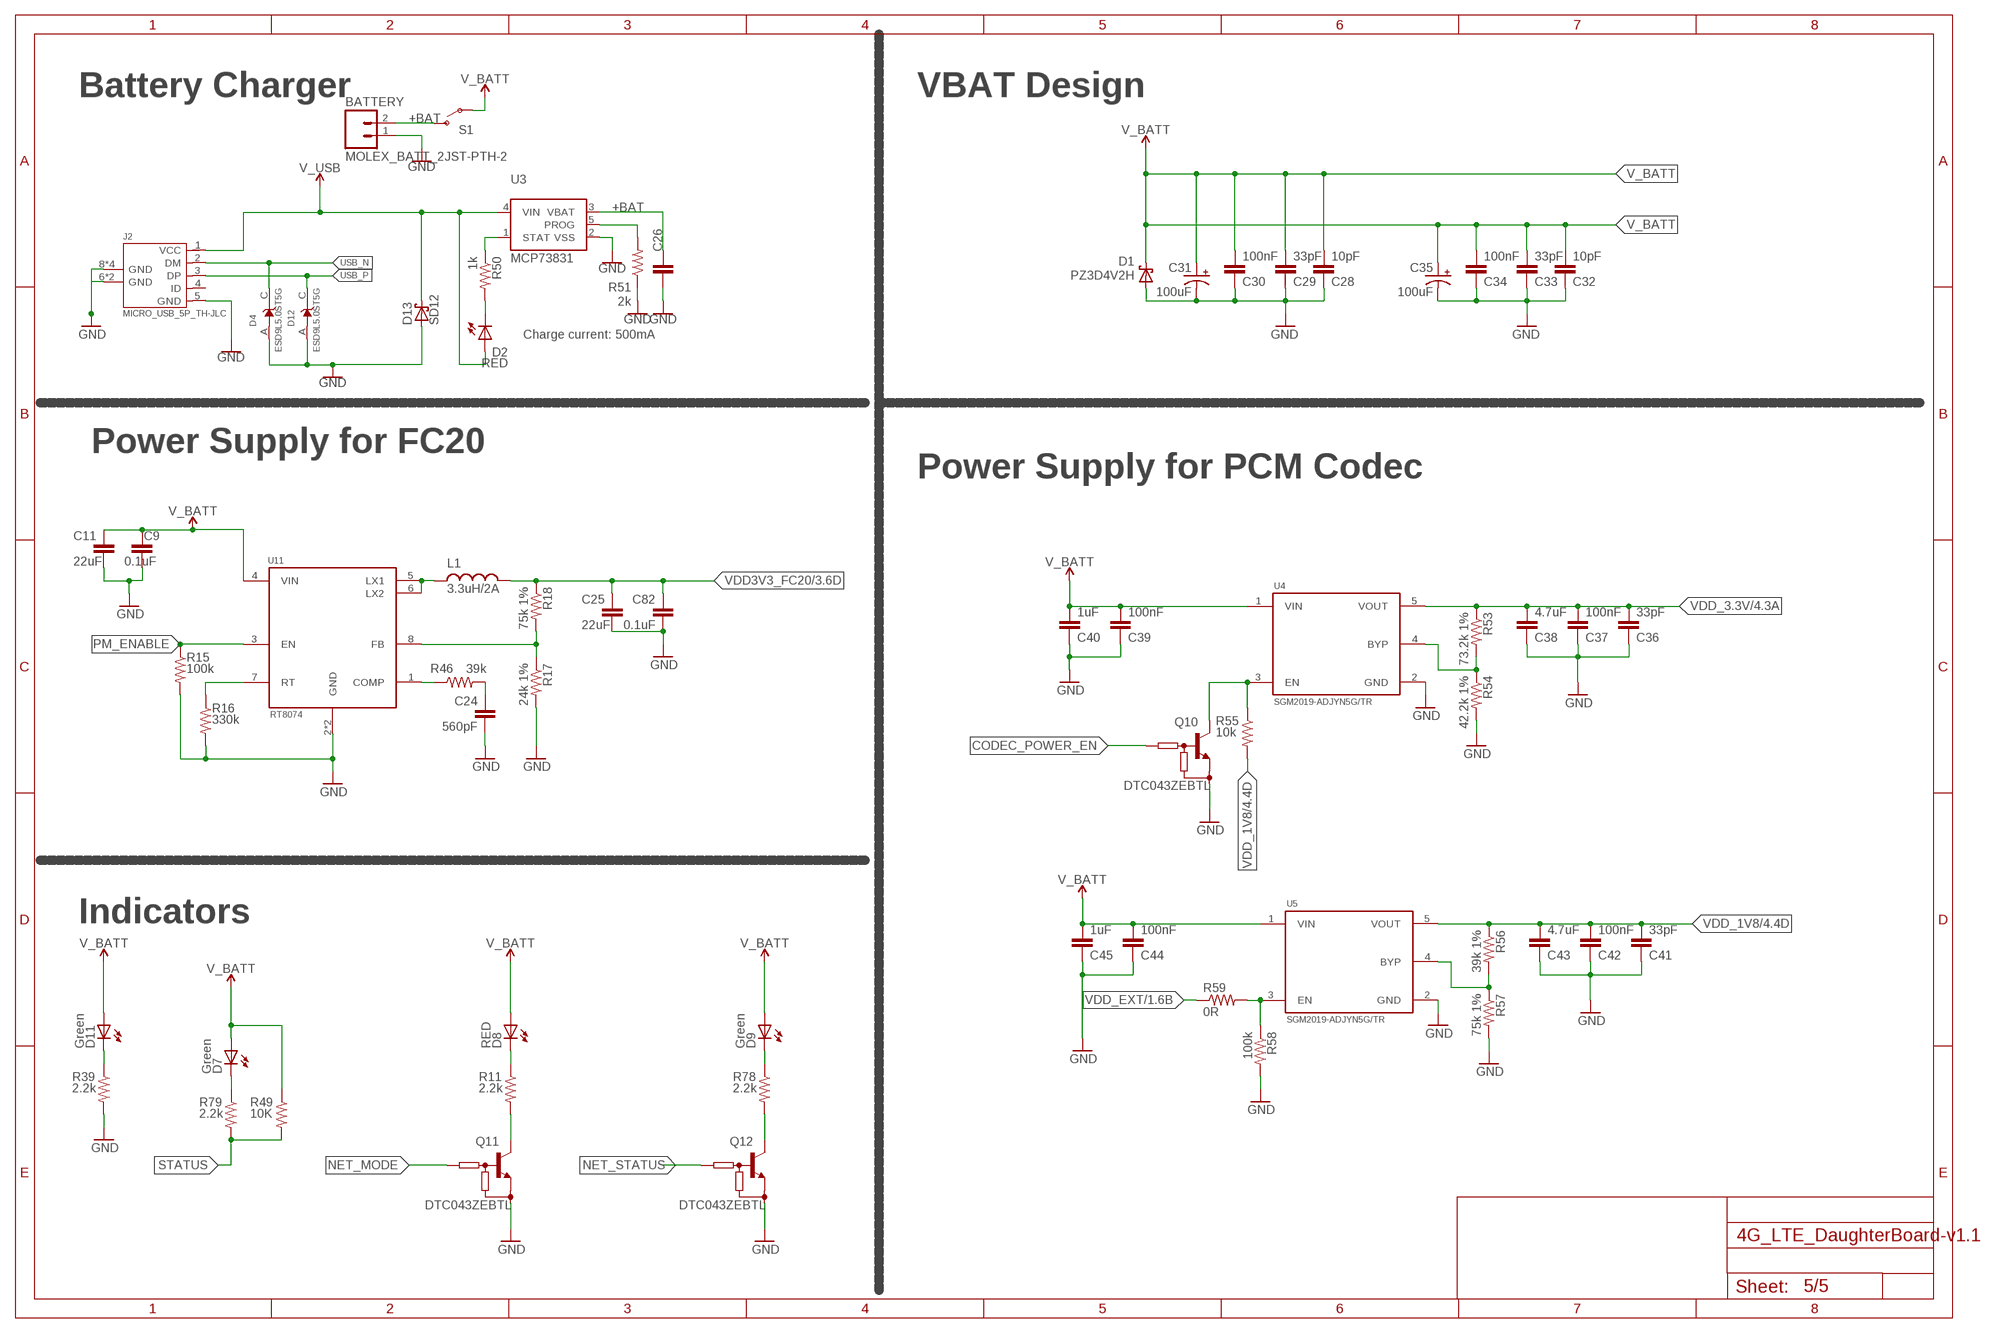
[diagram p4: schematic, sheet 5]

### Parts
BATTERY  MOLEX_BATT_2JST-PTH-2  [JST-2-PTH]
C9  0.1uF  CAP0402  [0402-CAP]
C11  22uF  CAP0805  [0805_CAP]
C24  560pF  CAP0402  [0402-CAP]
C25  22uF  CAP0805  [0805_CAP]
C26  4.7uF  CAP0402  [0402-CAP]
C28  10pF  CAP  [0603-CAP-L]
C29  33pF  CAP  [0603-CAP-L]
C30  100nF  CAP  [0603-CAP-L]
C31  100uF  CAP_TANT_AVX-B  [AVX-B]
C32  10pF  CAP  [0603-CAP-L]
C33  33pF  CAP  [0603-CAP-L]
C34  100nF  CAP  [0603-CAP-L]
C35  100uF  CAP_TANT_AVX-B  [AVX-B]
C36  33pF  CAP0402  [0402-CAP]
C37  100nF  CAP0402  [0402-CAP]
C38  4.7uF  CAP0402  [0402-CAP]
C39  100nF  CAP0402  [0402-CAP]
C40  1uF  CAP0402  [0402-CAP]
C41  33pF  CAP0402  [0402-CAP]
C42  100nF  CAP0402  [0402-CAP]
C43  4.7uF  CAP0402  [0402-CAP]
C44  100nF  CAP0402  [0402-CAP]
C45  1uF  CAP0402  [0402-CAP]
C82  0.1uF  CAP0402  [0402-CAP]
D1  PZ3D4V2H  DIODE_SCHOTTKEY  [SOD323]
D2  RED  LED0603  [0603-LED]
D4  ESD9L5.0ST5G  [SOD923]
D7  Green  LED0603  [0603-LED]
D8  RED  LED0603  [0603-LED]
D9  Green  LED0603  [0603-LED]
D11  Green  LED0603  [0603-LED]
D12  ESD9L5.0ST5G  [SOD923]
D13  SD12  DIODE_SCHOTTKEY  [SOD323]
J2  MICRO_USB_5P_TH-JLC  [B-SMD-5P-0.65SLOT]
L1  3.3uH/2A  IND4018  [IND4018]
Q10  DTC043ZEBTL  DIGITAL_TRANSISTOR-SC89  [SC89]
Q11  DTC043ZEBTL  DIGITAL_TRANSISTOR-SC89  [SC89]
Q12  DTC043ZEBTL  DIGITAL_TRANSISTOR-SC89  [SC89]
R11  2.2k  RES0402  [0402-RES]
R15  100k  RES0402  [0402-RES]
R16  330k  RES0402  [0402-RES]
R17  24k 1%  RES0402  [0402-RES]
R18  75k 1%  RES0402  [0402-RES]
R39  2.2k  RES0402  [0402-RES]
R46  39k  RES0402  [0402-RES]
R49  10K  RES0402  [0402-RES]
R50  1k  RES0402  [0402-RES]
R51  2k  RES0402  [0402-RES]
R53  73.2k 1%  RES0402  [0402-RES]
R54  42.2k 1%  RES0402  [0402-RES]
R55  10k  RES0402  [0402-RES]
R56  39k 1%  RES0402  [0402-RES]
R57  75k 1%  RES0402  [0402-RES]
R58  100k  RES0402  [0402-RES]
R59  0R  RES0402  [0402-RES]
R78  2.2k  RES0402  [0402-RES]
R79  2.2k  RES0402  [0402-RES]
S1  SS12D11  [SWITCH_SPDT_PTH_90D_13X9.2MM]
U3  MCP73831  [SOT23-5]
U4  SGM2019-ADJYN5G/TR  [SOT23-5(SOT95P280X145-5N)]
U5  SGM2019-ADJYN5G/TR  [SOT23-5(SOT95P280X145-5N)]
U11  RT8074  [SOP-8-150MIL(SOIC127P600X175-8T200)]

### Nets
$$$29: R17.1 R18.2 U11.8(FB)
+BAT: BATTERY.2 C26.1 S1.2(O) U3.3(VBAT)
CODEC_POWER_EN: Q10.1(B) ; also sheet 1
GND: BATTERY.1 C9.1 C11.2 C24.1 C25.2 C26.2 C28.1 C29.1 C30.1 C31.- C32.1 C33.1 C34.1 C35.- C36.1 C37.1 C38.1 C39.1 C40.1 C41.1 C42.1 C43.1 C44.1 C45.1 C82.1 D1.A D4.A D12.A D13.A J2.5(GND) J2.6(GND) J2.7(GND) J2.8(GND) J2.9(GND) J2.10(GND) J2.11(GND) Q10.2(E) Q11.2(E) Q12.2(E) R15.2 R16.2 R17.2 R39.2 R51.1 R54.2 R57.2 R58.2 U3.2(VSS) U4.2(GND) U5.2(GND) U11.2(GND) U11.9(GND) ; also sheet 1,2,3,4
N$13: R46.1 U11.1(COMP)
N$20: D8.C R11.1
N$22: C24.2 R46.2
N$23: D2.C R50.2
N$24: R50.1 U3.1(STAT)
N$25: R51.2 U3.5(PROG)
N$27: Q11.3(C) R11.2
N$28: R16.1 U11.7(RT)
N$30: L1.1 U11.5(LX1) U11.6(LX2)
N$31: R53.2 R54.1 U4.4(BYP)
N$32: Q10.3(C) R55.1 U4.3(EN)
N$33: R56.2 R57.1 U5.4(BYP)
N$34: R58.1 R59.2 U5.3(EN)
N$62: Q12.3(C) R78.2
N$63: D9.C R78.1
N$65: D11.C R39.1
N$67: D7.C R79.1
NET_MODE: Q11.1(B) ; also sheet 2
NET_STATUS: Q12.1(B) ; also sheet 2
PM_ENABLE: R15.1 U11.3(EN) ; also sheet 2
STATUS: R49.2 R79.2 ; also sheet 2
USB_N [USB_Data]: D4.C J2.2(DM) ; also sheet 2
USB_P [USB_Data]: D12.C J2.3(DP) ; also sheet 2
V_BATT: C9.2 C11.1 C28.2 C29.2 C30.2 C31.+ C32.2 C33.2 C34.2 C35.+ C39.2 C40.2 C44.2 C45.2 D1.C D7.A D8.A D9.A D11.A R49.1 S1.3(P) U4.1(VIN) U5.1(VIN) U11.4(VIN) ; also sheet 2
V_USB: D2.A D13.C J2.1(VCC) U3.4(VIN) ; also sheet 2
VDD3V3_FC20: C25.1 C82.2 L1.2 R18.1 ; also sheet 3
VDD_1V8: C41.2 C42.2 C43.2 R55.2 R56.1 U5.5(VOUT) ; also sheet 4
VDD_3.3V: C36.2 C37.2 C38.2 R53.1 U4.5(VOUT) ; also sheet 4
VDD_EXT: R59.1 ; also sheet 1,2,3
Unconnected: J2.4(ID)

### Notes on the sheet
- Battery Charger | VBAT Design
- Charge current: 500mA
- Power Supply for FC20
- Power Supply for PCM Codec
- Indicators

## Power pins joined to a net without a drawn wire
1: WIPHONE_DAUGHTERBOARD-FOOTPRINT1.1
12: WIPHONE_DAUGHTERBOARD-FOOTPRINT1.12
USIM2_VDD: U1.128(USIM2_VDD)
VDD_SDIO: U1.34(VDD_SDIO)
VPP: J1.C6(VPP)

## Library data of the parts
ANT1-ANT4 = WiPhone:U.FL2PIN
BATTERY = HackEDA V1.0:MOLEX_BATT_2: Header 2
C1-C11 C13-C30 C32-C34 C36-C83 C85-C90 = WiPhone:CAP: Capacitor.
C12 C31 C35 = HackEDA V1.0:CAP_TANT: Tantulum capacitor.
D1 D13 = WiPhone:DIODE_SCHOTTKEY: Schottky barrier diode
D2 D7-D9 D11 = HackEDA V1.0:LED: LED.
D3 D22 = WiPhone:LESD5D5.0CT1G
D4 D12 = WiPhone:ESD9L5.0ST5G
D5 = WiPhone:ESDA6V1-5W6: ESDA Series 5 Channel 6.1 V 50 pF SMT Uni-Directional Transil Array - SOT-323-6L; DESCRIPTION: ESDA Series 5 Channel 6.1 V 50 pF SMT Uni Directional Transil Array - SOT-323-6; MP: ESDA6V1-5W6; PACKAGE: SOT-323 STMicroelectronics
D6 = WiPhone:ESD9M5.0ST5G: Low Capacitance ESD Protection; Unidirectional; DESCRIPTION: Low Capacitance ESD Protection; Unidirectional; MP: ESD9M5.0ST5G; PACKAGE: SOD-923 ON Semiconductor
D10 D14 = WiPhone:ESD9X3.3ST5G: Low Capacitance ESD Protection; Unidirectional; DESCRIPTION: Low Capacitance ESD Protection; Unidirectional; MP: ESD9X3.3ST5G; PACKAGE: SOD-923 ON Semiconductor
FL1 = WiPhone:CHOKE: MURATA# DLP11SN900HL2L, D LP Series 90 Ohm Impedanc e 20 % 150 mA DCR 1.5 Ohm SMT Common Mode Choke
J1 = WiPhone:XUNPU-SMN-303
J2 = WiPhone:MICRO_USB_5P_TH: MICRO USB B SMD R/A
J3 = WiPhone:PJ-342-SMT_3.5MM
K1 = WiPhone:BUTTON: Momentary Tactile Switch
L1-L4 = WiPhone:IND: Inductor.
Q1-Q4 Q10-Q12 = WiPhone:DIGITAL_TRANSISTOR
Q6 = WiPhone:TRANS_NPN: NPN transistor Current controlled devices typically used to amplify current or used as a switch.
R1-R86 R89-R92 = WiPhone:RES: Resistor.
S1 = WiPhone:SS12D11: Single Pole, Double Throw (SPDT) Switch
TP1 TP2 = WiPhone:TEST-POINT: Test Points
U1 = HackEDA V1.0:EC25: IoT/M2M-optimized LTE Cat4 Module 50Mbps/150Mbps UART/USB2.0/PCM/USIM/SDIO 850MHz/900MHz/1800MHz/1900MHz 3.8V Surface...
U2 = HackEDA V1.0:FC20: No description set
U3 = WiPhone:MCP73831: Miniature single cell, fully integrated Li-Ion, Li-polymer charge management controller http://ww1.microchip.com/downloads/en/DeviceDoc/21984a.pdf IC-09995
U4 U5 = WiPhone:SGM2019-ADJYN5G/TR
U6 = HackEDA V1.0:TXS0104EPWR: 4-Bit Bidirectional Voltage-Level Translator for Open-Drain and Push-Pull Applications 14-TSSOP -40 to 85; AVAILABILITY: Unavailable; DESCRIPTION: 4-Bit Bidirectional Voltage-Level Translator for Open-Drain and Push-Pull Applications 14-TSSOP -40 to 85; MF: Texas Instruments; MP: TXS0104EPWR; PACKAGE: TSSOP-14 Texas Instruments; PRICE: None
U7 = WiPhone:ALC5616: Ultra-Low Power Audio CODEC for Mobile Devices, QFN-32 Source: Datasheet; DESCRIPTION: Ultra-Low Power Audio CODEC for Mobile Devices, QFN-32; MANUFACTURER_PART_NUMBER: ALC5616
U11 = WiPhone:RT8074
WIPHONE_DAUGHTERBOARD-FOOTPRINT1 = WiPhone:WIPHONE_DAUGHTERBOARD

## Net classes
1 USB_Data: width 0.261 mm, drill 0.305 mm, clearance 0.203 mm
2 SDIO3.0: width 0.235 mm, drill 0.305 mm, clearance 0.305 mm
